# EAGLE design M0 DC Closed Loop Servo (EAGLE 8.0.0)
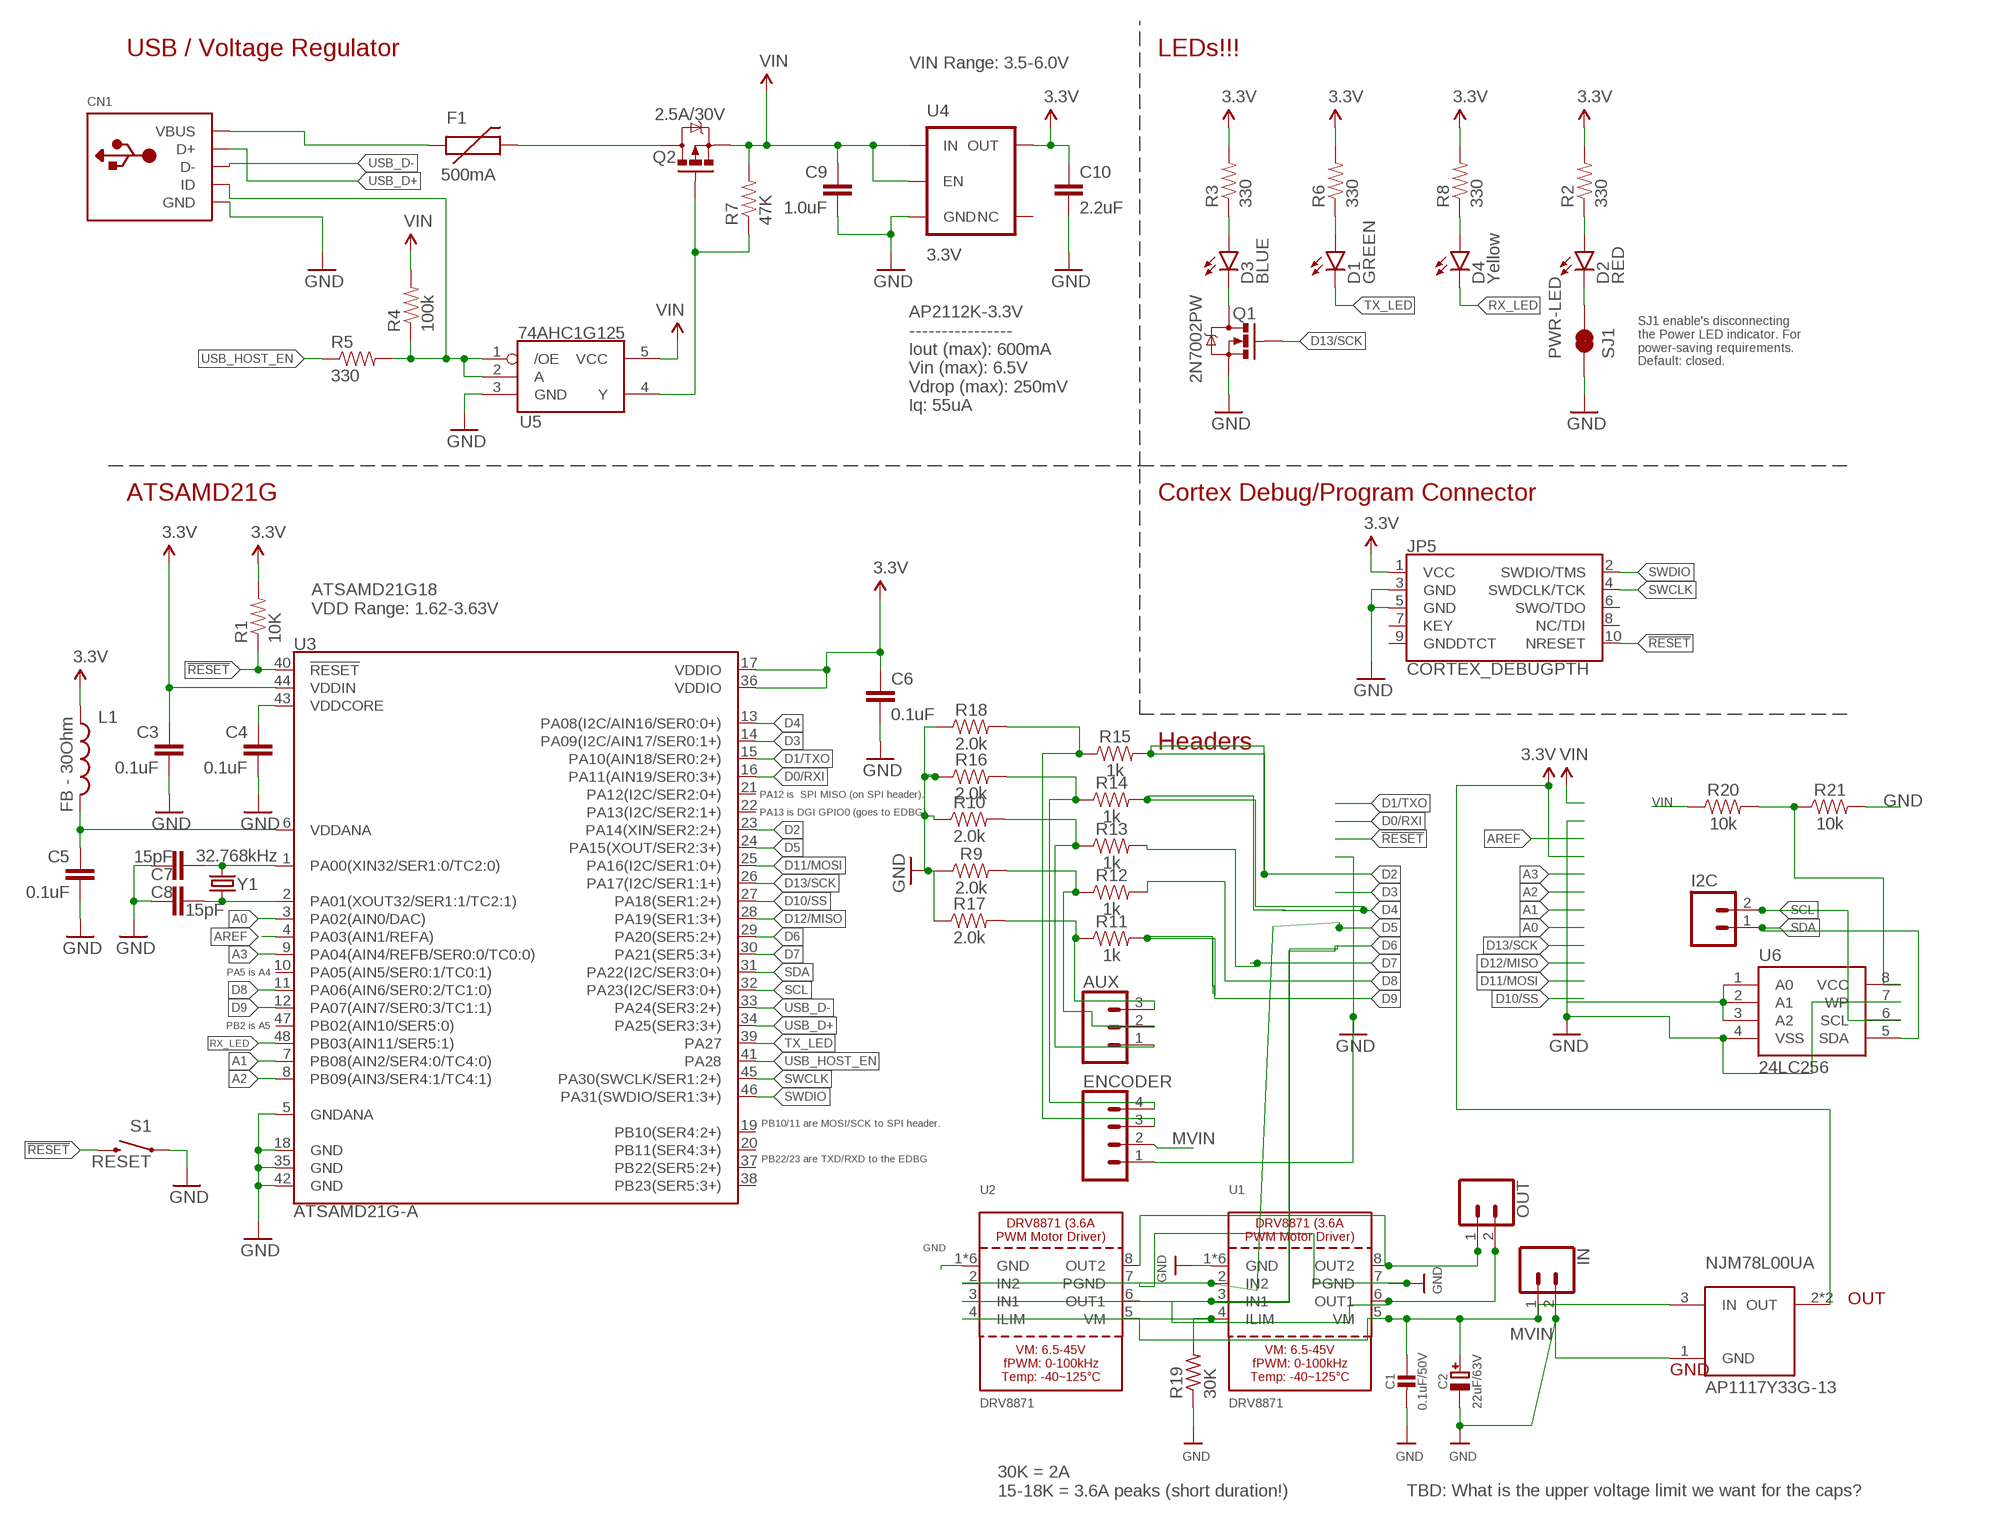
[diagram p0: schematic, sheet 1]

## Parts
AUX  CONN_03LONGPADS  [1X03_LONGPADS]
C1  0.1uF/50V  CAP_CERAMIC0805-NOOUTLINE  [0805-NO]
C2  22uF/63V  CAP_ELECTROLYTICPANASONIC_D  [PANASONIC_D]
C3  0.1uF  0.1UF-16V(+-10%)(0402)  [0402-CAP]
C4  0.1uF  0.1UF-16V(+-10%)(0402)  [0402-CAP]
C5  0.1uF  0.1UF-16V(+-10%)(0402)  [0402-CAP]
C6  0.1uF  0.1UF-16V(+-10%)(0402)  [0402-CAP]
C7  15pF  15PF-50V(+-5%)(0402)  [0402-CAP]
C8  15pF  15PF-50V(+-5%)(0402)  [0402-CAP]
C9  1.0uF  1.0UF-25V-+80/-20(0805)"  [0805-CAP]
C10  2.2uF  2.2UF-10V-20%(0603)  [0603-CAP]
CN1  USBMINIB  [USB-MINIB]
D1  GREEN  LED-GREEN0603  [LED-0603]
D2  RED  LED-RED0603  [LED-0603]
D3  BLUE  LED-BLUE0603  [LED-0603]
D4  Yellow  LED-YELLOW0603  [LED-0603]
ENCODER  CONN_04JST-PTH-VERT  [JST-4-PTH-VERT]
F1  500mA  PTCSMD  [PTC-1206]
I2C  M021X02_NO_SILK  [1X02_NO_SILK@1]
IN  CONN_02PTH3  [1X02_LONGPADS]
JP5  CORTEX_DEBUGPTH  [2X5-PTH-1.27MM]
L1  FB - 30Ohm  INDUCTOR0603  [0603]
NJM78L00UA  AP1117Y33G-13  [SOT89]
OUT  CONN_02PTH3  [1X02_LONGPADS]
Q1  2N7002PW  MOSFET-NCHANNEL2N7002PW  [SOT323]
Q2  2.5A/30V  MOSFET-PCHANNELDMG2307L  [SOT23-3]
R1  10K  10KOHM-1/10W-1%(0603)0603  [0603-RES]
R2  330  330OHM1/10W1%(0603)  [0603-RES]
R3  330  330OHM1/10W1%(0603)  [0603-RES]
R4  100k  100KOHM-1/10W-1%(0603)  [0603-RES]
R5  330  330OHM1/10W1%(0603)  [0603-RES]
R6  330  330OHM1/10W1%(0603)  [0603-RES]
R7  47K  47KOHM1/10W1%(0603)  [0603-RES]
R8  330  330OHM1/10W1%(0603)  [0603-RES]
R9  2.0k  2.0KOHM-0603-1/10W-5%  [0603]
R10  2.0k  2.0KOHM-0603-1/10W-5%  [0603]
R11  1k  1KOHM-0603-1/10W-1%  [0603]
R12  1k  1KOHM-0603-1/10W-1%  [0603]
R13  1k  1KOHM-0603-1/10W-1%  [0603]
R14  1k  1KOHM-0603-1/10W-1%  [0603]
R15  1k  1KOHM-0603-1/10W-1%  [0603]
R16  2.0k  2.0KOHM-0603-1/10W-5%  [0603]
R17  2.0k  2.0KOHM-0603-1/10W-5%  [0603]
R18  2.0k  2.0KOHM-0603-1/10W-5%  [0603]
R19  30K  FLIPFLOP-RES  [0805-THM]
R20  10k  10KOHM-0603-1/10W-1%  [0603]
R21  10k  10KOHM-0603-1/10W-1%  [0603]
S1  RESET  SWITCH-MOMENTARY-2SMD-4.6X2.8MM  [TACTILE_SWITCH_SMD_4.6X2.8MM]
SJ1  PWR-LED  JUMPER-PAD-2-NC_BY_TRACENO_SILK  [PAD-JUMPER-2-NC_BY_TRACE_NO_SILK]
U1  DRV8871  [HSOP8]
U2  DRV8871  [HSOP8]
U3  ATSAMD21G-A  [TQFP-48]
U4  3.3V  V_REG_AP2112K-3.3V  [SOT23-5]
U5  74AHC1G125  [SOT23-5]
U6  24LC256  EEPROM-I2CSMD  [SO08]
Y1  32.768kHz  CRYSTAL3.2X1.5MM  [CRYSTAL-SMD-3.2X1.5MM]

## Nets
3.3V: C3.1 C6.1 C10.1 JP5.1(VCC) L1.1 NJM78L00UA.2(OUT) NJM78L00UA.2@1(OUT) R1.2 R2.2 R3.2 R6.2 R8.2 U3.17(VDDIO) U3.36(VDDIO) U3.44(VDDIN) U4.5(OUT)
!RESET: JP5.10(NRESET) R1.1 S1.3 S1.4 U3.40(!RESET!)
A0: U3.3(PA02(AIN0/DAC))
A1: U3.7(PB08(AIN2/SER4:0/TC4:0))
A2: U3.8(PB09(AIN3/SER4:1/TC4:1))
A3: U3.9(PA04(AIN4/REFB/SER0:0/TC0:0))
AREF: U3.4(PA03(AIN1/REFA))
D0/RXI: U3.16(PA11(AIN19/SER0:3+))
D1/TXO: U3.15(PA10(AIN18/SER0:2+))
D2: R15.2 U3.23(PA14(XIN/SER2:2+))
D3: U3.14(PA09(I2C/AIN17/SER0:1+))
D4: R14.2 U3.13(PA08(I2C/AIN16/SER0:0+))
D5: U1.2(IN2) U2.2(IN2) U3.24(PA15(XOUT/SER2:3+))
D6: U1.3(IN1) U2.3(IN1) U3.29(PA20(SER5:2+))
D7: R13.2 U3.30(PA21(SER5:3+))
D8: R12.2 U3.11(PA06(AIN6/SER0:2/TC1:0))
D9: R11.2 U3.12(PA07(AIN7/SER0:3/TC1:1))
D10/SS: U3.27(PA18(SER1:2+))
D11/MOSI: U3.25(PA16(I2C/SER1:0+))
D12/MISO: U3.28(PA19(SER1:3+))
D13/SCK: Q1.1(G) U3.26(PA17(I2C/SER1:1+))
ENCODER: ENCODER.3 R15.1 R18.2
GND: C1.2 C2.- C3.2 C4.2 C5.2 C6.2 C7.1 C8.2 C9.2 C10.2 CN1.GND ENCODER.1 IN.2 JP5.3(GND) JP5.5(GND) NJM78L00UA.1(GND) Q1.2(S) R9.1 R10.1 R16.1 R17.1 R18.1 R19.1 R21.2 S1.1 S1.2 SJ1.1 U1.1(GND) U1.7(PGND) U1.GND U1.P$1(GND) U1.P$2(GND) U1.P$3(GND) U1.P$4(GND) U2.1(GND) U2.7(PGND) U2.GND U2.P$1(GND) U2.P$2(GND) U2.P$3(GND) U2.P$4(GND) U3.5(GNDANA) U3.18(GND) U3.35(GND) U3.42(GND) U4.2(GND) U5.3(GND) U6.1(A0) U6.2(A1) U6.3(A2) U6.4(VSS) U6.7(WP)
MVIN: C1.1 C2.+ ENCODER.2 IN.1 NJM78L00UA.3(IN) U1.5(VM) U2.5(VM)
N$1: CN1.VBUS F1.1
N$2: C7.2 U3.1(PA00(XIN32/SER1:0/TC2:0)) Y1.P$2
N$3: D3.C Q1.3(D)
N$4: C8.1 U3.2(PA01(XOUT32/SER1:1/TC2:1)) Y1.P$1
N$5: D2.A R2.1
N$6: D3.A R3.1
N$7: F1.2 Q2.3(D)
N$8: CN1.ID R4.1 R5.2 U5.1(/OE) U5.2(A)
N$9: Q2.1(G) R7.1 U5.4(Y)
N$10: D1.A R6.1
N$11: D4.A R8.1
N$12: D2.C SJ1.2
N$14: AUX.3 R11.1 R17.2
N$15: R20.2 R21.1 U6.8(VCC)
N$16: AUX.2 R9.2 R12.1
N$17: AUX.1 R10.2 R13.1
N$18: ENCODER.4 R14.1 R16.2
N$20: R19.2 U1.4(ILIM) U2.4(ILIM)
OUT1: OUT.2 U1.6(OUT1) U2.6(OUT1)
OUT2: OUT.1 U1.8(OUT2) U2.8(OUT2)
RX_LED: D4.C U3.48(PB03(AIN11/SER5:1))
SCL: I2C.2 U3.32(PA23(I2C/SER3:0+)) U6.6(SCL)
SDA: I2C.1 U3.31(PA22(I2C/SER3:0+)) U6.5(SDA)
SWCLK: JP5.4(SWDCLK/TCK) U3.45(PA30(SWCLK/SER1:2+))
SWDIO: JP5.2(SWDIO/TMS) U3.46(PA31(SWDIO/SER1:3+))
TX_LED: D1.C U3.39(PA27)
USB_D+: CN1.D+ U3.34(PA25(SER3:3+))
USB_D-: CN1.D- U3.33(PA24(SER3:2+))
USB_HOST_EN: R5.1 U3.41(PA28)
VDDANA: C5.1 L1.2 U3.6(VDDANA)
VDDCORE: C4.1 U3.43(VDDCORE)
VIN: C9.1 Q2.2(S) R4.2 R7.2 R20.1 U4.1(IN) U4.3(EN) U5.5(VCC)
Unconnected: JP5.6(SWO/TDO) JP5.7(KEY) JP5.8(NC/TDI) JP5.9(GNDDTCT) U3.10(PA05(AIN5/SER0:1/TC0:1)) U3.19(PB10(SER4:2+)) U3.20(PB11(SER4:3+)) U3.21(PA12(I2C/SER2:0+)) U3.22(PA13(I2C/SER2:1+)) U3.37(PB22(SER5:2+)) U3.38(PB23(SER5:3+)) U3.47(PB02(AIN10/SER5:0)) U4.4(NC)

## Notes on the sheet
- USB / Voltage Regulator | LEDs!!!
- VIN Range: 3.5-6.0V
- AP2112K-3.3V
  ----------------
  Iout (max): 600mA 
  Vin (max): 6.5V
  Vdrop (max): 250mV
  Iq: 55uA
- SJ1 enable's disconnecting
  the Power LED indicator. For
  power-saving requirements.
  Default: closed.
- ATSAMD21G | Cortex Debug/Program Connector
- ATSAMD21G18
  VDD Range: 1.62-3.63V
- Headers
- PA12 is  SPI MISO (on SPI header).
- PA13 is DGI GPIO0 (goes to EDBG).
- PA5 is A4
- PB2 is A5
- PB10/11 are MOSI/SCK to SPI header.
- PB22/23 are TXD/RXD to the EDBG
- OUT
- GND
- 30K = 2A
  15-18K = 3.6A peaks (short duration!)
- TBD: What is the upper voltage limit we want for the caps?

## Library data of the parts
AUX = SparkFun-Connectors:CONN_03: Multi connection point. Often used as Generic Header-pin footprint for 0.1 inch spaced/style header connections On any of the 0.1 inch spaced packages, you can populate with these: Break Away Headers - Straight (PRT-00116) Break Away Male Headers - Right Angle (PRT-00553) Female Headers (PRT-00115)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
C1 = microbuilder:CAP_CERAMIC: Ceramic Capacitors
C2 = microbuilder:CAP_ELECTROLYTIC: Electrolytic Capacitors
C3-C6 = SparkFun-Capacitors:0.1UF-16V(+-10%)(0402); PROD_ID: CAP-12416
C7 C8 = samd21-temp:15PF-50V(+-5%)(0402); PROD_ID: CAP-13063
C9 = SparkFun-Capacitors:1.0UF-25V-+80/-20(0805): CAP-11625; PROD_ID: CAP-11625
C10 = SparkFun-Capacitors:2.2UF-10V-20%(0603): CAP-07888; PROD_ID: CAP-07888
CN1 = adafruit:USB: USB Connectors USBMINIB - Surface Mount Female Mini-B USB Connector 4UConnector: 06564 By microbuilder.eu Thru-hole RA Female Mini-B USB Connector 4UConnector: 18732 By ladyada.net
D1 = SparkFun-LED:LED-GREEN: Various green LEDs; PROD_ID: DIO-00821
D2 = SparkFun-LED:LED-RED: Assorted Red LEDs; PROD_ID: DIO-00819
D3 = SparkFun-LED:LED-BLUE: Blue LEDs for production use; PROD_ID: DIO-08575
D4 = SparkFun-LED:LED-YELLOW: Yellow SMD LEDs; PROD_ID: DIO-09003
ENCODER = SparkFun-Connectors:CONN_04: Multi connection point. Often used as Generic Header-pin footprint for 0.1 inch spaced/style header connections On any of the 0.1 inch spaced packages, you can populate with these: Break Away Headers - Straight (PRT-00116) Break Away Male Headers - Right Angle (PRT-00553) Female Headers (PRT-00115)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; PROD_ID: CONN-13251
F1 = SparkFun-PowerIC:PTC: Resettable Fuse PTC; PROD_ID: RES-11150
I2C = SparkFun-Connectors:M02: Standard 2-pin 0.1" header. Use with
IN OUT = SparkFun-Connectors:CONN_02: Multi connection point. Often used as Generic Header-pin footprint for 0.1 inch spaced/style header connections
JP5 = samd21-temp:CORTEX_DEBUG: Cortex Debug Connector Datasheet
L1 = SparkFun-Passives:INDUCTOR: Inductors; PROD_ID: RES-07859
NJM78L00UA = AP1117Y33G-13:AP1117Y33G-13
Q1 = SparkFun-DiscreteSemi:MOSFET-NCHANNEL: Common NMOSFET Parts MFG P/NStore IDProd ID FDD8780TRANS-09984 SI7820DNTRANS-11055 FDS6630AIC-08089 2N7002PWTRANS-11151 FQP30N06L COM-10213TRANS-10060 BSS123LT1GTRANS-08345 BSS138TRANS-00830 BS170 2N7000; PROD_ID: TRANS-11151
Q2 = SparkFun-DiscreteSemi:MOSFET-PCHANNEL: Generic PMOSFET IRLML2244 - TRANS-11153 (SOT-23 -20V -4.3A) (1.Gate 2.Source 3.Drain) FQP27P06 - COM-10349 (TO-220 -60V -27A) (1.Gate 2.Source 3.Drain); PROD_ID: TRANS-11308
R1 = SparkFun-Resistors:10KOHM-1/10W-1%(0603): RES-00824; PROD_ID: RES-00824
R2 R3 R5 R6 R8 = SparkFun-Resistors:330OHM1/10W1%(0603): RES-00818; PROD_ID: RES-00818
R4 = SparkFun-Resistors:100KOHM-1/10W-1%(0603): RES-07828; PROD_ID: RES-07828
R7 = SparkFun-Resistors:47KOHM1/10W1%(0603): RES-07871; PROD_ID: RES-07871
R9 R10 R16-R18 = SparkFun-Resistors:2.0KOHM: 2kΩ resistor; PROD_ID: RES-08296
R11-R15 = SparkFun-Resistors:1KOHM: 1kΩ resistor; PROD_ID: RES-07856
R19 = adafruit:FLIPFLOP-RES: Flip Flop resistor
R20 R21 = SparkFun-Resistors:10KOHM: 10kΩ resistor; PROD_ID: RES-00824
S1 = samd21-temp:SWITCH-MOMENTARY-2: Various NO switches- pushbuttons, reed, etc; PROD_ID: SWCH-13065
SJ1 = SparkFun-Passives:JUMPER-PAD-2-NC_BY_TRACE
U1 U2 = microbuilder:DRV8871: DRV8871 - 3.6A PWM Motor Driver
U3 = samd21-temp:ATSAMD21G: Atmel SAMD21G SMART ARM-Based Microcontroller The Atmel ® | SMART ™ SAM D21 is a series of low-power microcontrollers using the 32-bit ARM ® Cortex ® -M0+ processor, and ranging from 32- to 64-pins with up to 256KB Flash and 32KB of SRAM. The SAM D21 devices operate at a maximum frequency of 48MHz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; PROD_ID: IC-13064
U4 = SparkFun-PowerIC:V_REG_AP2112: AP2112 - 600mA CMOS LDO Regulator w/ Enable The AP2112 is CMOS process low dropout linear regulator with enable function, the regulator delivers a guaranteed 600mA (min.) continuous load current. Features Output Voltage Accuracy: ±1.5% Output Current: 600mA (Min.) Foldback Short Current Protection: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; PROD_ID: VREG-12457
U5 = SparkFun-DigitalIC:74AHC1G125: Single bus buffer gate with 3-state output; PROD_ID: IC-11920
U6 = SparkFun-IC-Memory:EEPROM-I2C: I2C EEPROMs, 24LC256 and others 24LC256 Series 256 kb I2C 2 Wire (32 k x 8 Bit) 2.5 V Serial EEPROM SMD - SOIC-8 Datasheet SparkFun Products SparkFun UDB5 - PIC UAV Development Board (GPS-11703); PROD_ID: IC-09714
Y1 = samd21-temp:CRYSTAL: Various standard crystals. Proven footprints.; PROD_ID: XTAL-13062

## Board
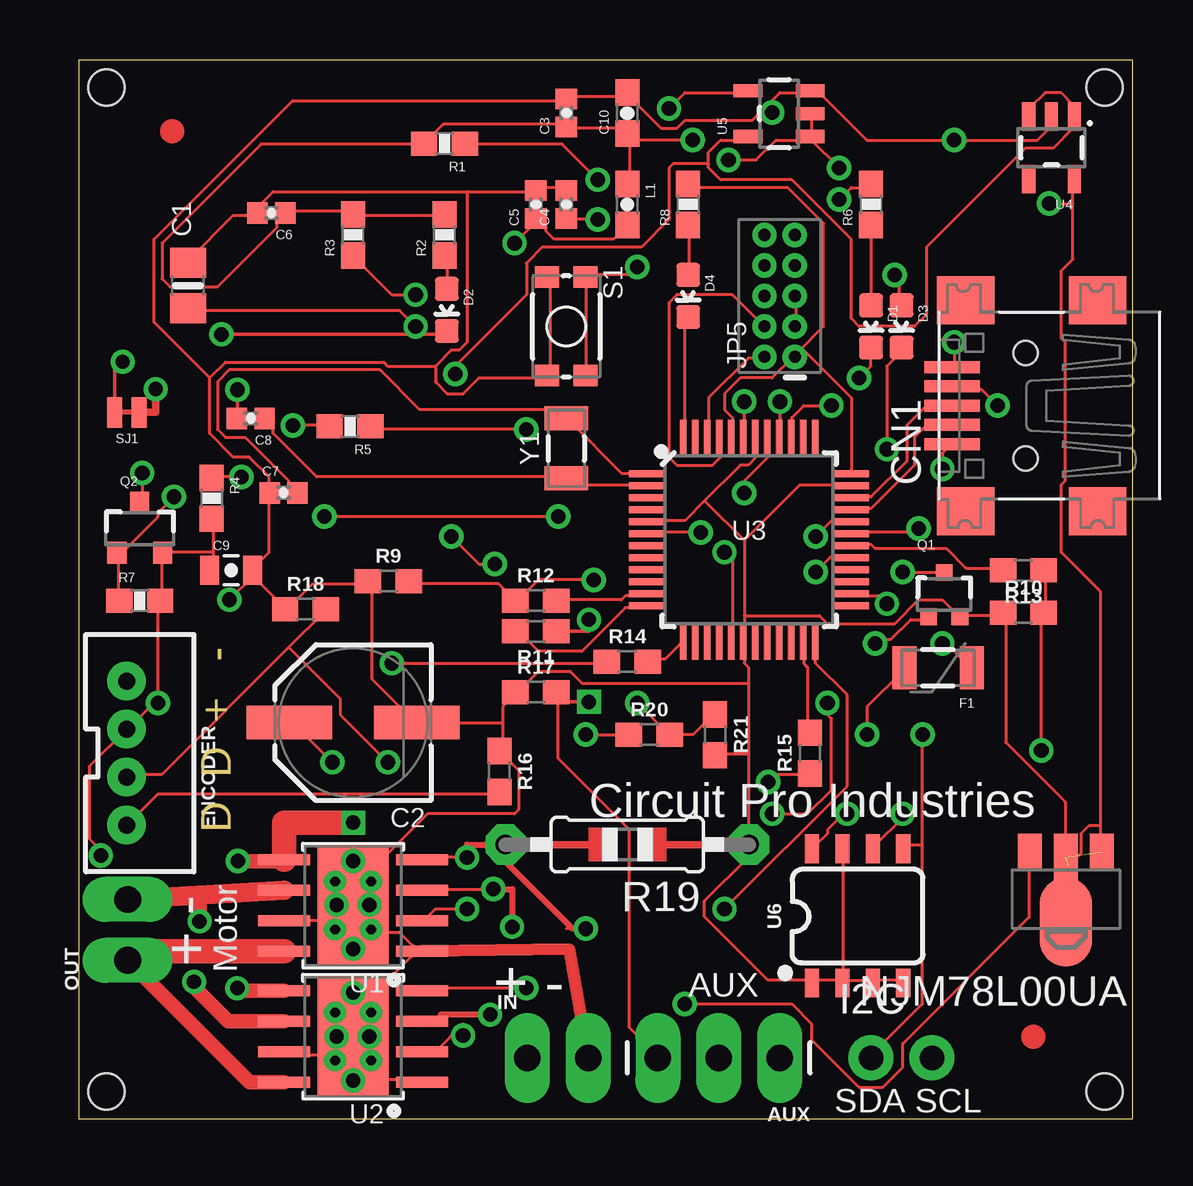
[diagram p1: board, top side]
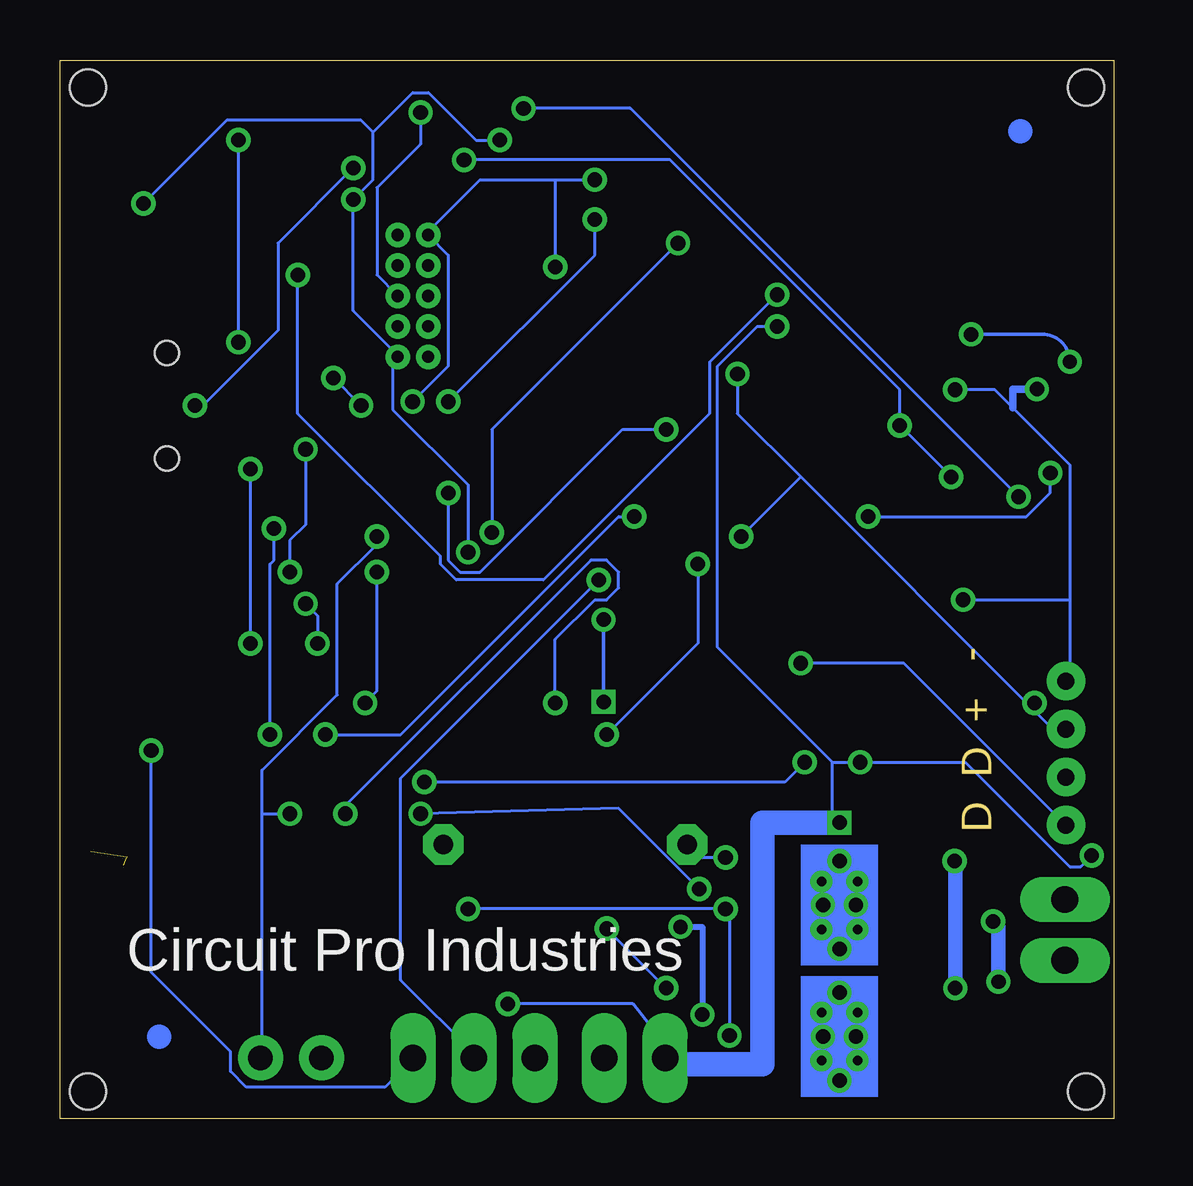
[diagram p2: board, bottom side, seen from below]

Size 43.92 x 44.12 mm. Coordinates in mm from the lower left corner, seen from the top.
Outline: 0,0 43.92,0 43.92,44.12 0,44.12 0,0
Copper layers (1*16): Top 0.035mm / dielectric 1.5mm / Bottom 0.035mm
Design rules "default *": minimum track width 5mil, minimum drill 24mil, track to track 8mil, track to pad 8mil, pad to pad 8mil, via to via 8mil, smd to smd 8mil, copper to edge 40mil, drill to drill 8mil, minimum pad ring 10mil, minimum via ring 8mil, stop-mask expansion 4mil, vias tented up to drill 0mil, thermal gap 10mil
Holes 1.5 mm at 42.75,42.98 1.14,42.98 1.14,1.14 42.75,1.14

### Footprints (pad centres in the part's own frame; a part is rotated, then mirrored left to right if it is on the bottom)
1X03_LONGPADS = drill 1.118 pad 1.88 long: 1 0,0; 2 2.54,0; 3 5.08,0
0805-NO = smd 1.24 x 1.5: 1 -0.95,0; 2 0.95,0
PANASONIC_D = smd 3.556 x 1.4: + 2.654,0; - -2.654,0
0402-CAP = smd 0.85 x 0.9: 1 -0.58,0; 2 0.58,0
0805-CAP = smd 0.8 x 1.2: 1 -0.9,0; 2 0.9,0
0603-CAP = smd 1.1 x 1: 1 -0.85,0; 2 0.85,0
USB-MINIB = smd 0.5 x 2.308: D+ 0,4.064; D- -0.8,4.064; GND 1.6,4.064; ID 0.8,4.064; VBUS -1.6,4.064 | smd 2 x 2.4: GND1 -4.4,-2; GND2 -4.4,3.5; GND3 4.4,3.5; GND4 4.4,-2 | hole 1: -2.2,1; 2.2,1
LED-0603 = smd 1 x 1: A 0,-0.877; C 0,0.877
JST-4-PTH-VERT = drill 0.7 pad 1.6: 1 -3,-0.55; 2 -1,-0.55; 3 1,-0.55; 4 3,-0.55
PTC-1206 = smd 1 x 1.8: 1 -1.4,0; 2 1.4,0
1X02_NO_SILK@1 = drill 1.016 pad 1.88: 1 0,0; 2 2.54,0
1X02_LONGPADS = drill 1.118 pad 1.88 long: 1 0,0; 2 2.54,0
2X5-PTH-1.27MM = drill 0.508 pad 1: 1 -2.54,-0.635; 2 -2.54,0.635; 3 -1.27,-0.635; 4 -1.27,0.635; 5 0,-0.635; 6 0,0.635; 7 1.27,-0.635; 8 1.27,0.635; 9 2.54,-0.635; 10 2.54,0.635
0603 = smd 1.1 x 1: 1 -0.85,0; 2 0.85,0
SOT89 = smd 1 x 1.5: 1 -1.499,-1.981; 3 1.499,-1.981 | smd 1 x 2: 2 0,-1.727 | smd 2.2 x 3.7: 2@1 0,0.94
SOT323 = smd 0.7 x 0.7: 1 -0.65,-0.925; 2 0.65,-0.925; 3 0,0.925
SOT23-3 = smd 0.8 x 0.9: 1 -0.95,-1; 2 0.95,-1; 3 0,1.1
0603-RES = smd 1.1 x 1: 1 -0.85,0; 2 0.85,0
0805-THM = drill 0.813 pad 1.676 octagon: 1 -5.08,0; 2 5.08,0
TACTILE_SWITCH_SMD_4.6X2.8MM = smd 0.9 x 1: 1 -2.05,-0.8; 2 2.05,-0.8; 3 2.05,0.8; 4 -2.05,0.8
PAD-JUMPER-2-NC_BY_TRACE_NO_SILK = smd 0.635 x 1.27: 1 -0.508,0; 2 0.508,0
HSOP8 = smd 0.45 x 2.15: 1 -1.905,-2.875; 2 -0.635,-2.875; 3 0.635,-2.875; 4 1.905,-2.875; 5 1.905,2.875; 6 0.635,2.875; 7 -0.635,2.875; 8 -1.905,2.875 | smd 4.9 x 2.95: GND 0,0 | drill 0.4: P$1 -1,0.75; P$2 -1,-0.75; P$3 1,-0.75; P$4 1,0.75
TQFP-48 = smd 1.5 x 0.28: 1 -4.25,2.75; 2 -4.25,2.25; 3 -4.25,1.75; 4 -4.25,1.25; 5 -4.25,0.75; 6 -4.25,0.25; 7 -4.25,-0.25; 8 -4.25,-0.75; 9 -4.25,-1.25; 10 -4.25,-1.75; 11 -4.25,-2.25; 12 -4.25,-2.75; 25 4.25,-2.75; 26 4.25,-2.25; 27 4.25,-1.75; 28 4.25,-1.25; 29 4.25,-0.75; 30 4.25,-0.25; 31 4.25,0.25; 32 4.25,0.75; 33 4.25,1.25; 34 4.25,1.75; 35 4.25,2.25; 36 4.25,2.75 | smd 0.28 x 1.5: 13 -2.75,-4.25; 14 -2.25,-4.25; 15 -1.75,-4.25; 16 -1.25,-4.25; 17 -0.75,-4.25; 18 -0.25,-4.25; 19 0.25,-4.25; 20 0.75,-4.25; 21 1.25,-4.25; 22 1.75,-4.25; 23 2.25,-4.25; 24 2.75,-4.25; 37 2.75,4.25; 38 2.25,4.25; 39 1.75,4.25; 40 1.25,4.25; 41 0.75,4.25; 42 0.25,4.25; 43 -0.25,4.25; 44 -0.75,4.25; 45 -1.25,4.25; 46 -1.75,4.25; 47 -2.25,4.25; 48 -2.75,4.25
SOT23-5 = smd 0.55 x 1.2: 1 -0.95,-1.3; 2 0,-1.3; 3 0.95,-1.3; 4 0.95,1.3; 5 -0.95,1.3
SO08 = smd 0.6 x 1.2: 1 -1.905,-2.8; 2 -0.635,-2.8; 3 0.635,-2.8; 4 1.905,-2.8; 5 1.905,2.8; 6 0.635,2.8; 7 -0.635,2.8; 8 -1.905,2.8
CRYSTAL-SMD-3.2X1.5MM = smd 1 x 1.8: P$1 -1.25,0; P$2 1.25,0

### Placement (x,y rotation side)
AUX  29.21,2.54 180 top
C1  4.55,34.72 90 top
C2  11.43,16.51 180 top
C3  20.32,41.91 90 top
C4  20.32,38.1 90 top
C5  19.05,38.1 90 top
C6  8.03,37.74 180 top
C7  8.53,26.09 0 top
C8  7.16,29.18 180 top
C9  6.35,22.86 0 top
C10  22.86,41.91 90 top
CN1  40.46,29.72 90 top
D1  33.02,33.02 180 top
D2  15.34,33.71 180 top
D3  34.29,33.02 180 top
D4  25.4,34.29 180 top
ENCODER  2.54,15.24 270 top
F1  35.81,18.8 180 top
I2C  33.02,2.54 0 top
IN  18.69,2.54 0 top
JP5  29.21,34.29 90 top
L1  22.86,38.1 270 top
NJM78L00UA  41.15,9.14 180 top
OUT  2.03,6.6 90 top
Q1  36.07,21.84 0 top
Q2  2.54,24.59 0 top
R1  15.24,40.64 180 top
R2  15.24,36.83 90 top
R3  11.43,36.83 90 top
R4  5.54,25.86 270 top
R5  11.3,28.85 180 top
R6  33.02,38.1 90 top
R7  2.54,21.59 0 top
R8  25.4,38.1 90 top
R9  12.9,22.4 0 top
R10  39.37,21.08 0 top
R11  19.05,20.32 180 top
R12  19.05,21.59 0 top
R13  39.37,22.86 180 top
R14  22.86,19.05 0 top
R15  30.48,15.24 90 top
R16  17.53,14.48 270 top
R17  19.05,17.78 0 top
R18  9.45,21.23 0 top
R19  22.86,11.43 180 top
R20  23.77,16 0 top
R21  26.52,16 270 top
S1  20.32,33.02 270 top
SJ1  2.01,29.44 180 top
U1  11.43,8.89 90 top
U2  11.43,3.43 90 top
U3  27.94,24.13 0 top
U4  40.54,40.46 180 top
U5  29.18,41.88 90 top
U6  32.46,8.46 0 top
U$7  [CIRCLE-1MM-3R]  39.78,3.43 0 top
U$8  [CIRCLE-1MM-3R]  3.89,41.15 0 top
Y1  20.32,27.94 90 top

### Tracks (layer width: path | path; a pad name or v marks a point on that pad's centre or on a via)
3.3V  (via drill 0.61)  (1 unrouted)
  Top 0.127: 41.44,38.14 41.44,35.83 40.95,35.33 40.95,32.52 41.11,32.36 41.11,26.58 40.95,26.42 40.95,23.61 42.6,21.96 42.6,12.22 | 41.44,38.14 41.44,39.13 U4.5 | 42.6,11.23 42.6,12.22 | R2.2 15.19,37.64 11.56,37.64 R3.2 11.39,37.81 8.75,37.81 C6.1 8.59,37.64 8.26,37.31 8.26,37.15 5.78,34.67 3.8,34.67 3.47,35 3.47,36.49 7.59,40.62 14.36,40.62 R1.2 14.53,40.78 15.19,41.44 20.31,41.44 C3.1 20.47,41.27 22.62,41.27 22.78,41.11 C10.1 | 22.95,40.78 22.95,40.95 C10.1 | 22.95,40.78 22.95,38.96 L1.1 | 30.05,32.03 29.88,31.86 JP5.1 | 30.05,32.03 31.04,33.02 31.04,37.31 29.55,38.8 25.43,38.8 R8.2 | v31.7,38.3 32.19,38.8 33.02,38.8 R6.2 | v26.91,23.61 27.24,23.28 27.24,19.98 U3.17 | 30.05,32.03 30.21,32.03 32.19,30.05 32.19,26.91 U3.36 | 30.05,32.03 JP5.1 | U3.44 27.24,28.4 27.24,29.22 26.91,29.55 26.91,30.21 27.57,30.87 28.89,30.87 29.72,31.7 JP5.1 | v25.59,40.78 22.95,40.78 | 22.95,40.78 C10.1 | v40.45,38.14 41.44,38.14 | 42.6,12.22 42.1,12.22 41.77,11.89 41.77,11.06 41.27,10.57 41.27,8.26 NJM78L00UA.2@1
  Bottom 0.127: v26.91,23.61 26.91,26.42 30.05,29.55 30.05,31.53 29.88,31.7 JP5.1 29.88,31.86 31.7,33.68 v31.7,38.3 30.87,39.13 30.87,41.11 | v25.59,40.78 26.58,40.78 28.56,42.76 29.22,42.76 30.87,41.11 | v40.45,38.14 36.98,41.6 31.37,41.6 30.87,41.11
!RESET  (via drill 0.61)
  Top 0.127: S1.3 21.13,31.04 21.13,35 S1.4 21.13,35.17 22.95,35.17 v23.28,35.5 | v21.63,39.13 20.14,40.62 16.18,40.62 R1.1 | v29.22,29.88 29.22,28.4 U3.40
  Bottom 0.127: 23.28,39.13 26.42,39.13 28.56,36.98 JP5.10 27.74,35.99 27.74,31.37 v29.22,29.88 | 23.28,39.13 v21.63,39.13 | 23.28,39.13 v23.28,35.5
D2
  Top 0.127: R15.2 30.38,16.18 30.38,18.82 30.21,18.99 30.21,19.81 U3.23
D4
  Top 0.127: R14.2 23.77,19.15 24.43,19.15 25.09,19.81 U3.13
D5  (via drill 0.61)
  Top 0.127: v26.91,8.75 32.03,13.87 32.03,17.67 30.71,18.99 30.71,19.81 U3.24 | v16.18,8.75 14.86,8.75 14.36,8.26 U1.2 | v16.02,3.48 16.02,3.96 14.86,2.81 14.36,2.81 U2.2
  Bottom 0.127: v26.91,8.75 v16.18,8.75 16.02,8.59 v16.02,3.48
D6  (via drill 0.6, 0.61)
  Top 0.127: v30.71,22.78 31.37,23.44 32.03,23.44 U3.29 | v31.2,17.34 31.2,16.84 31.37,16.68 31.37,13.7 30.38,12.71 v28.89,12.71 | v17.27,9.58 14.36,9.58 U1.3
  Top 0.254: v17.27,9.58 18.06,9.58 v18.06,8 | v17.14,4.34 15.09,4.34 15.09,4.12 14.3,4.12 U2.3
  Bottom 0.127: v30.71,22.78 30.71,17.83 v31.2,17.34 | v28.89,12.71 20.64,12.94 v17.27,9.58
  Bottom 0.254: v18.06,8 17.14,8 v17.14,4.34
D7
  Top 0.127: R13.2 38.47,22.95 36.98,22.95 36.16,23.77 33.19,23.77 33.02,23.94 32.19,23.94 U3.30
D8
  Top 0.127: R12.2 19.98,21.63 22.62,21.63 22.78,21.79 23.61,21.79 U3.11
D9
  Top 0.127: R11.2 18.33,20.31 19.15,19.48 20.97,19.48 22.78,21.3 23.61,21.3 U3.12
D13/SCK  (via drill 0.61)
  Top 0.127: v33.19,19.81 33.35,19.98 33.85,19.98 34.67,20.8 35.33,20.8 Q1.1 | v33.68,21.46 33.35,21.79 32.19,21.79 U3.26
  Bottom 0.127: v33.19,19.81 33.19,20.97 v33.68,21.46
ENCODER  (via drill 0.61)
  Top 0.127: 8.75,19.65 3.47,14.36 2.15,14.36 ENCODER.3 | 8.75,19.65 10.24,21.13 R18.2 | v28.73,14.03 29.06,14.36 30.38,14.36 R15.1 | v12.88,14.86 10.9,16.84 10.9,17.5 8.75,19.65
  Bottom 0.127: v28.73,14.03 13.7,14.03 v12.88,14.86
GND  (via drill 0.6, 0.61)  (1 unrouted)
  Top 0.127: 26.09,25.76 27.57,27.24 27.9,27.24 28.23,27.57 28.23,28.23 U3.42 | 26.09,25.76 25.26,24.93 23.77,24.93 U3.5 | 27.74,24.11 27.74,20.97 | 27.74,20.97 27.74,19.98 U3.18 27.74,19.81 27.74,18.99 27.9,18.82 27.9,18.16 | 26.09,25.76 27.74,24.11 | 27.74,24.11 30.05,26.42 32.03,26.42 U3.35 | 27.74,20.97 30.87,20.97 31.2,20.64 34.01,20.64 35,21.63 35.99,21.63 36.65,20.97 Q1.2 36.82,20.97 38.47,20.97 R10.1 38.63,20.97 38.63,15.68 41.11,13.21 41.11,10.9 | 27.9,18.16 27.9,15.19 | 27.9,15.19 27.9,11.56 R19.1 27.9,11.39 27.9,10.9 26.09,9.08 26.09,8.42 28.73,5.78 30.54,5.78 U6.1 30.71,5.78 31.7,5.78 U6.2 31.86,5.78 | JP5.3 29.88,33.02 29.88,34.18 JP5.5 | 28.4,41.94 28.07,41.6 25.26,41.6 24.93,41.27 24.27,41.27 22.95,42.6 C10.2 22.78,42.6 20.47,42.6 C3.2 20.31,42.43 8.91,42.43 3.14,36.65 3.14,33.19 5.45,30.87 | 28.4,41.94 29.22,42.76 30.38,42.76 U5.3 30.54,42.76 30.87,42.76 32.85,40.78 v36.49,40.78 39.95,40.78 40.45,41.27 40.45,41.6 U4.2 | v36.49,32.36 36.49,31.37 CN1.GND | 28.4,41.94 v28.89,41.94 | S1.1 19.65,35 19.65,31.04 S1.2 19.48,30.87 16.68,30.87 16.02,30.21 15.35,30.21 14.86,30.71 14.86,31.37 | C4.2 20.31,38.8 19.15,38.8 C5.2 18.99,38.63 16.18,38.63 | C1.2 4.62,35.83 6.44,37.64 7.43,37.64 C6.2 7.59,37.81 7.59,38.14 8.09,38.63 16.18,38.63 | 14.86,31.37 15.52,32.03 15.85,32.03 16.18,32.36 16.18,38.63 | v6.6,30.38 6.6,29.22 C8.2 | 11.39,8.59 11.56,8.75 U1.GND | 11.39,8.59 10.73,7.92 U1.P$1 10.57,7.92 10.24,8.26 U1.7 | 11.39,9.08 11.56,8.91 U1.GND | 11.39,9.08 10.73,9.74 U1.P$4 | 11.39,8.59 12.05,7.92 U1.P$2 12.22,7.76 13.37,7.76 13.87,7.26 U1.1 13.87,6.77 12.22,5.12 12.22,4.46 U2.P$3 12.05,4.29 11.39,3.63
  Top 0.127: 11.39,8.59 U1.GND | 11.39,9.08 12.05,9.74 U1.P$3 12.22,9.91 12.22,10.4 14.53,12.71 18.16,12.71 18.33,12.88 18.33,14.53 17.67,15.19 R16.1 17.67,15.35 17.67,16.51 | 11.39,9.08 U1.GND | 7.92,26.09 7.92,23.61 7.26,22.95 C9.2 | 7.26,22.62 7.1,22.78 C9.2 | 7.26,22.62 8.59,21.3 R18.1 8.75,21.3 9.74,22.29 12.05,22.29 R9.1 12.22,22.29 12.22,18.33 14.03,16.51 C2.- 17.67,16.51 | 17.67,16.51 17.67,17.17 18.16,17.67 R17.1 18.33,17.83 19.15,18.66 20.47,18.66 20.97,18.16 27.9,18.16 | 7.26,22.62 v6.27,21.63 | 7.26,22.62 C9.2 | 14.86,31.37 12.88,31.37 12.71,31.53 6.11,31.53 5.45,30.87 | 5.45,30.87 5.45,28.56 6.44,27.57 7.1,27.57 7.92,26.75 7.92,26.09 | 7.92,26.09 C7.1 | 11.39,3.14 11.56,3.3 U2.GND | 11.39,3.14 10.73,2.48 U2.P$1 10.57,2.48 10.4,2.64 8.59,2.64 U2.7 | 11.39,3.63 11.56,3.47 U2.GND | 11.39,3.63 10.73,4.29 U2.P$4 | 11.39,3.14 12.05,2.48 U2.P$2 12.22,2.31 12.88,1.65 14.2,1.65 U2.1 | 11.39,3.14 U2.GND | 11.39,3.63 U2.GND | U6.4 34.34,5.78 33.19,5.78 U6.3 33.02,5.78 31.86,5.78 | 27.9,15.19 26.58,15.19 R21.2 | 31.86,5.78 31.86,11.23 U6.7
  Top 0.305: SJ1.1 3.2,29.44 v3.2,30.4
  Top 0.508: IN.2 20.45,7.06 U1.1
  Bottom 0.127: v36.49,40.78 v36.49,32.36 | v28.89,41.94 28.89,40.62 30.71,38.8 30.71,35.17 29.88,34.34 JP5.5 | v6.6,30.38 4.95,30.38 4.2,29.63 1.82,27.24 1.82,21.63 | 1.82,21.63 1.82,18.49 1.98,18.33 ENCODER.1 | v6.27,21.63 1.82,21.63
  Bottom 0.305: v3.2,30.4 4.2,30.4 4.2,29.63
MVIN  (via drill 0.6, 0.61)
  Top 0.127: v14.03,33.02 13.37,33.68 4.62,33.68 C1.1 | v25.26,4.79 29.72,4.79 30.54,3.96 30.54,3.3 32.52,1.32 33.52,1.32 34.34,2.15 34.34,3.14 39.62,8.42 39.62,11.06 NJM78L00UA.3 | v10.57,14.86 8.91,16.51 C2.+ | v6.6,5.45 8.42,5.45 U2.5 | v0.91,10.97 0.91,11.2 0.46,11.66 0.46,14.71 ENCODER.2
  Top 0.61: U2.5 6.72,5.33 v6.6,5.45 | v6.63,10.74 8.5,10.74 U1.5
  Top 1.016: v11.43,12.34 8.55,12.34 U1.5
  Bottom 0.127: v14.03,33.02 14.86,33.02 16.51,31.37 16.51,19.65 11.72,14.86 | 11.72,14.86 11.72,12.71 v11.43,12.34 | v25.26,4.79 20.04,4.79 19.14,3.66 IN.1 | 11.72,14.86 v10.57,14.86 6.17,14.86 1.83,10.52 1.37,10.52 v0.91,10.97
  Bottom 0.61: v6.6,5.45 6.6,10.72 v6.63,10.74
  Bottom 1.016: v11.43,12.34 14.63,12.34 14.63,2.29 17.78,2.29 IN.1
N$1  (via drill 0.61)
  Top 0.127: v35.99,19.81 36.16,19.81 37.15,18.82 F1.1 | v35.99,27.08 35.99,27.74 36.32,28.07 CN1.VBUS
  Bottom 0.127: v35.99,27.08 v35.99,19.81
N$2
  Top 0.127: C7.2 9.08,26.09 8.75,26.42 8.75,26.58 6.93,28.4 6.11,28.4 5.78,28.73 5.78,30.71 6.27,31.2 12.55,31.2 14.2,29.55 19.98,29.55 20.31,29.22 Y1.P$2 20.47,29.06 22.62,26.91 23.61,26.91 U3.1
N$3  (via drill 0.61)
  Top 0.127: v34.34,22.78 35.99,22.78 Q1.3 | v33.68,27.9 33.68,31.37 34.34,32.03 D3.C
  Bottom 0.127: v34.34,22.78 34.34,24.11 33.68,24.77 v33.68,27.9
N$4
  Top 0.127: C8.1 7.76,29.06 8.09,28.73 8.09,28.56 9.91,26.75 20.31,26.75 Y1.P$1 20.47,26.58 20.64,26.42 23.61,26.42 U3.2
N$5
  Top 0.127: D2.A 15.35,34.67 15.35,35.83 R2.1
N$6  (via drill 0.61)
  Top 0.127: v34.01,35.17 34.18,35 34.18,34.01 D3.A | v14.03,34.34 13.04,34.34 11.56,35.83 R3.1
  Bottom 0.127: v34.01,35.17 34.01,29.39 28.07,23.44 28.07,23.11 27.41,22.45 23.77,22.45 16.84,29.39 16.84,31.53 v14.03,34.34
N$7  (via drill 0.61)
  Top 0.127: v2.64,26.91 2.64,25.76 Q2.3 | v19.98,25.09 v10.24,25.09 | v32.85,16.02 32.85,17.17 34.34,18.66 F1.2
  Bottom 0.127: v2.64,26.91 2.64,26.09 3.63,25.09 v10.24,25.09 | v19.98,25.09 20.64,25.09 29.72,16.02 v32.85,16.02
N$8  (via drill 0.61)
  Top 0.127: U5.1 30.54,40.95 30.54,41.77 U5.2 | v6.77,26.75 5.61,26.75 R4.1 | v8.91,28.89 10.4,28.89 R5.2 | v27.08,39.95 28.23,39.95 29.06,40.78 30.38,40.78 U5.1 | v38.3,29.72 37.64,30.38 36.49,30.38 CN1.ID | v31.7,39.62 30.54,40.78 U5.1
  Bottom 0.127: v6.77,26.75 v8.91,28.89 8.91,30.38 18.49,39.95 v27.08,39.95 | v38.3,29.72 37.97,29.72 34.84,32.85 34.84,36.49 v31.7,39.62
N$9  (via drill 0.61)
  Top 0.127: 1.65,23.44 1.65,21.63 R7.1 | v24.6,42.1 25.26,42.76 27.74,42.76 U5.4 | v3.96,25.92 3.3,25.26 3.3,25.09 1.65,23.44 | 1.65,23.44 Q2.1
  Bottom 0.127: v24.6,42.1 20.14,42.1 v3.96,25.92
N$10
  Top 0.127: R6.1 D1.A
N$11
  Top 0.127: D4.A 25.43,35.33 25.43,37.15 R8.1
N$12  (via drill 0.6)
  Top 0.152: D2.C 15.34,32.69 v5.94,32.69 | v1.83,31.55 1.5,31.55 SJ1.2
  Bottom 0.152: v5.94,32.69 2.97,32.69 arc90 v1.83,31.55
N$14  (via drill 0.6)
  Top 0.127: R17.2 19.98,17.67 19.98,15.02 22.95,12.05 22.95,3.8 24.11,2.64 AUX.3
  Top 0.152: R17.2 19.9,17.37 v21.26,17.37 | v21.26,20.8 21.26,20.32 R11.1
  Bottom 0.152: v21.26,17.37 v21.26,20.8
N$15  (via drill 0.61)
  Top 0.127: R21.1 26.42,16.84 25.59,16.02 24.77,16.02 R20.2 24.6,16.02 v23.28,17.34 | v32.03,12.71 31.86,12.71 31.2,12.05 31.2,11.89 30.71,11.39 U6.8
  Bottom 0.127: v32.03,12.71 32.03,13.04 21.79,23.28 21.13,23.28 20.64,22.78 20.64,22.12 21.13,21.63 21.63,21.63 23.28,19.98 v23.28,17.34
N$16  (via drill 0.61)
  Top 0.127: R9.2 13.87,22.29 17.5,22.29 18.16,21.63 R12.1 18.33,21.63 19.15,22.45 v21.46,22.45
  Bottom 0.127: v21.46,22.45 29.72,14.2 29.72,5.78 26.58,2.64 AUX.2
N$17  (via drill 0.61)
  Top 0.127: R13.1 40.28,22.78 40.28,21.13 R10.2 40.12,20.97 v40.12,15.35
  Bottom 0.127: v40.12,15.35 40.12,6.11 36.82,2.81 36.82,1.98 36.16,1.32 30.38,1.32 29.22,2.48 AUX.1
N$18  (via drill 0.61)
  Top 0.127: R16.2 17.5,13.54 3.3,13.54 2.15,12.38 ENCODER.4 | v13.04,18.99 21.96,18.99 R14.1
  Bottom 0.127: v13.04,18.99 8.75,18.99 2.15,12.38 ENCODER.4
N$19  (via drill 0.6)
  other vias: 11.43,5.26
N$20  (via drill 0.61)
  Top 0.127: v16.18,10.9 14.36,10.9 U1.4 | v18.66,5.45 14.36,5.45 U2.4 | 20.31,7.92 20.57,7.92 v21.13,7.92
  Top 0.254: v16.18,10.9 16.18,11.43 R19.2 17.78,10.72 20.57,7.92
  Bottom 0.127: 17.17,10.9 v16.18,10.9 | 17.67,11.39 R19.2 | v21.13,7.92 v18.66,5.45
N$21  (via drill 0.6)
  other vias: 12.12,8.92
N$22  (via drill 0.6)
  other vias: 10.74,8.92
N$23  (via drill 0.6)
  other vias: 11.43,7.09
N$24  (via drill 0.6)
  other vias: 11.43,10.74
N$25  (via drill 0.6)
  other vias: 12.12,3.43
N$26  (via drill 0.6)
  other vias: 10.74,3.43
N$27  (via drill 0.6)
  other vias: 11.43,1.6
OUT1  (via drill 0.6)
  Top 0.61: U2.6 6.22,4.06 4.8,5.49 v4.8,5.71 | v5.03,8.23 5.03,8.84 4.58,9.29
  Top 0.813: OUT.2 4.58,9.29 U1.6
  Bottom 0.61: v4.8,5.71 4.8,8 v5.03,8.23
OUT2
  Top 0.127: 7.92,1.65 8.42,1.65 U2.8
  Top 0.61: U2.8 7.11,1.52 OUT.1
  Top 1.016: OUT.1 2.41,6.99 U1.8
RX_LED
  Top 0.127: D4.C 25.26,33.35 25.26,28.4 U3.48
SCL  (via drill 0.61)
  Top 0.127: v30.71,24.27 31.37,24.93 32.03,24.93 U3.32 | v34.34,12.71 34.34,12.55 33.19,11.39 U6.6
  Bottom 0.127: v30.71,24.27 30.71,23.94 32.36,22.29 32.36,17.67 35.5,14.53 35.5,12.71 | 35.5,12.71 35.5,2.64 I2C.2 | 35.5,12.71 v34.34,12.71
SDA  (via drill 0.61)
  Top 0.127: v35,24.6 34.84,24.43 32.19,24.43 U3.31 | 35.17,11.39 35.17,4.79 33.02,2.64 I2C.1 | 35.17,11.39 v35.17,16.02 | 35.17,11.39 34.51,11.39 U6.5
  Bottom 0.127: v35,24.6 35,23.28 35.17,23.11 v35.17,16.02
SWCLK
  Top 0.127: U3.45 26.75,28.23 26.75,27.57 26.42,27.24 24.93,27.24 24.6,27.57 24.6,34.01 24.93,34.34 27.24,34.34 JP5.4
SWDIO
  Top 0.127: U3.46 26.25,28.4 26.25,30.05 27.9,31.7 28.56,31.7 JP5.2
TX_LED  (via drill 0.61)
  Top 0.127: D1.C 33.02,31.37 v32.52,30.87 | v31.37,29.72 30.21,29.72 29.72,29.22 29.72,28.4 U3.39
  Bottom 0.127: v31.37,29.72 v32.52,30.87
USB_D+
  Top 0.127: CN1.D+ 35.33,29.72 34.51,28.89 34.51,27.41 33.02,25.92 32.19,25.92 U3.34
USB_D-
  Top 0.127: U3.33 32.19,25.43 33.02,25.43 34.84,27.24 34.84,28.4 35.33,28.89 36.32,28.89 CN1.D-
USB_HOST_EN  (via drill 0.61)
  Top 0.127: v18.66,28.73 12.22,28.73 R5.1 | v27.74,26.09 27.74,26.58 28.73,27.57 28.73,28.23 U3.41
  Bottom 0.127: v18.66,28.73 20.47,28.73 26.42,22.78 27.24,22.78 27.74,23.28 v27.74,26.09
VDDANA  (via drill 0.61)
  Top 0.127: 19.15,37.48 19.48,37.15 19.48,36.98 19.81,36.65 22.29,36.65 22.78,37.15 L1.2 | v25.92,24.43 23.77,24.43 U3.6 | 19.15,37.48 v18.16,36.49 | 19.15,37.48 C5.1
  Bottom 0.127: v25.92,24.43 25.92,28.73 v18.16,36.49
VDDCORE  (via drill 0.61)
  Top 0.127: v21.63,37.48 20.47,37.48 C4.1 | v27.74,29.88 27.74,28.4 U3.43
  Bottom 0.127: v21.63,37.48 21.63,35.99 v27.74,29.88
VIN  (via drill 0.61)
  Top 0.127: 5.61,23.61 5.61,22.95 C9.1 | 5.61,23.61 5.61,24.93 R4.2 | 5.61,23.61 3.63,23.61 Q2.2 3.47,23.44 3.47,21.63 R7.2 3.3,21.46 3.3,17.5 3.14,17.34 | 2.15,16.34 3.14,17.34 | 26.25,39.79 26.25,39.62 26.75,39.13 29.72,39.13 32.19,36.65 32.19,33.35 32.52,33.02 34.84,33.02 35.33,33.52 35.33,36.32 39.46,40.45 40.62,40.45 41.44,41.27 41.44,41.6 U4.1 41.44,41.77 41.44,42.27 40.95,42.76 40.28,42.76 39.62,42.1 39.62,41.77 U4.3 | 26.25,39.79 26.25,40.28 26.75,40.78 27.74,40.78 U5.5 | v15.68,31.04 15.68,31.37 18.66,34.34 18.66,35.66 19.32,36.32 23.44,36.32 24.6,37.48 24.6,39.62 24.77,39.79 26.25,39.79 | v3.3,17.34 3.14,17.34 | v21.13,16.02 22.78,16.02 R20.1 | v17.34,23.11 16.68,23.11 v15.52,24.27
  Bottom 0.127: 2.15,16.34 2.64,16.34 3.47,17.17 | 13.04,26.75 15.68,29.39 v15.68,31.04 | 13.04,26.75 3.47,17.17 | 3.47,17.17 v3.3,17.34 | v21.13,16.02 17.34,19.81 v17.34,23.11 | 13.04,26.75 v15.52,24.27
(copper drawn outside any net)
  shapes: Bottom area x2

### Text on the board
Dimension: D D + -
tPlace: Circuit Pro Industries | + - | Motor | + - | AUX | SDA SCL
bPlace: Circuit Pro Industries

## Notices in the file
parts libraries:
SparkFun-Connectors: Licensing: Creative Commons ShareAlike 4.0 International - https://creativecommons.org/licenses/by-sa/4.0
microbuilder: This work is placed in the public domain, and may be freely used for commercial and non-commercial work with the following conditions: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
